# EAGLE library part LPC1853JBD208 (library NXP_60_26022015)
32-bit ARM Cortex-M3 MCU; up to 1 MB flash and 136 kB SRAM; Ethernet, two High-speed USB, LCD, EMC The LPC185x/3x/2x/1x are ARM Cortex-M3 based microcontrollers for embedded applications. The ARM Cortex-M3 is a next generation core that offers system enhancements such as low power consumption, enhanced debug features, and a high level of support block integration. The LPC185x/3x/2x/1x operate at CPU frequencies of up to 180 MHz. The ARM Cortex-M3 CPU incorporates a 3-stage pipeline and uses a Harvard architecture with separate local instruction and data buses as well as a third bus for peripherals. The ARM Cortex-M3 CPU also includes an internal prefetch unit that supports speculative branching. The LPC185x/3x/2x/1x include up to 1 MB of flash and 136 kB of on-chip SRAM, 16 kB of EEPROM memory, a quad SPI Flash Interface (SPIFI), a State Configurable Timer (SCT) subsystem, two High-speed USB controllers, Ethernet, LCD, an external memory controller, and multiple digital and analog peripherals. AAL Eindhoven MK
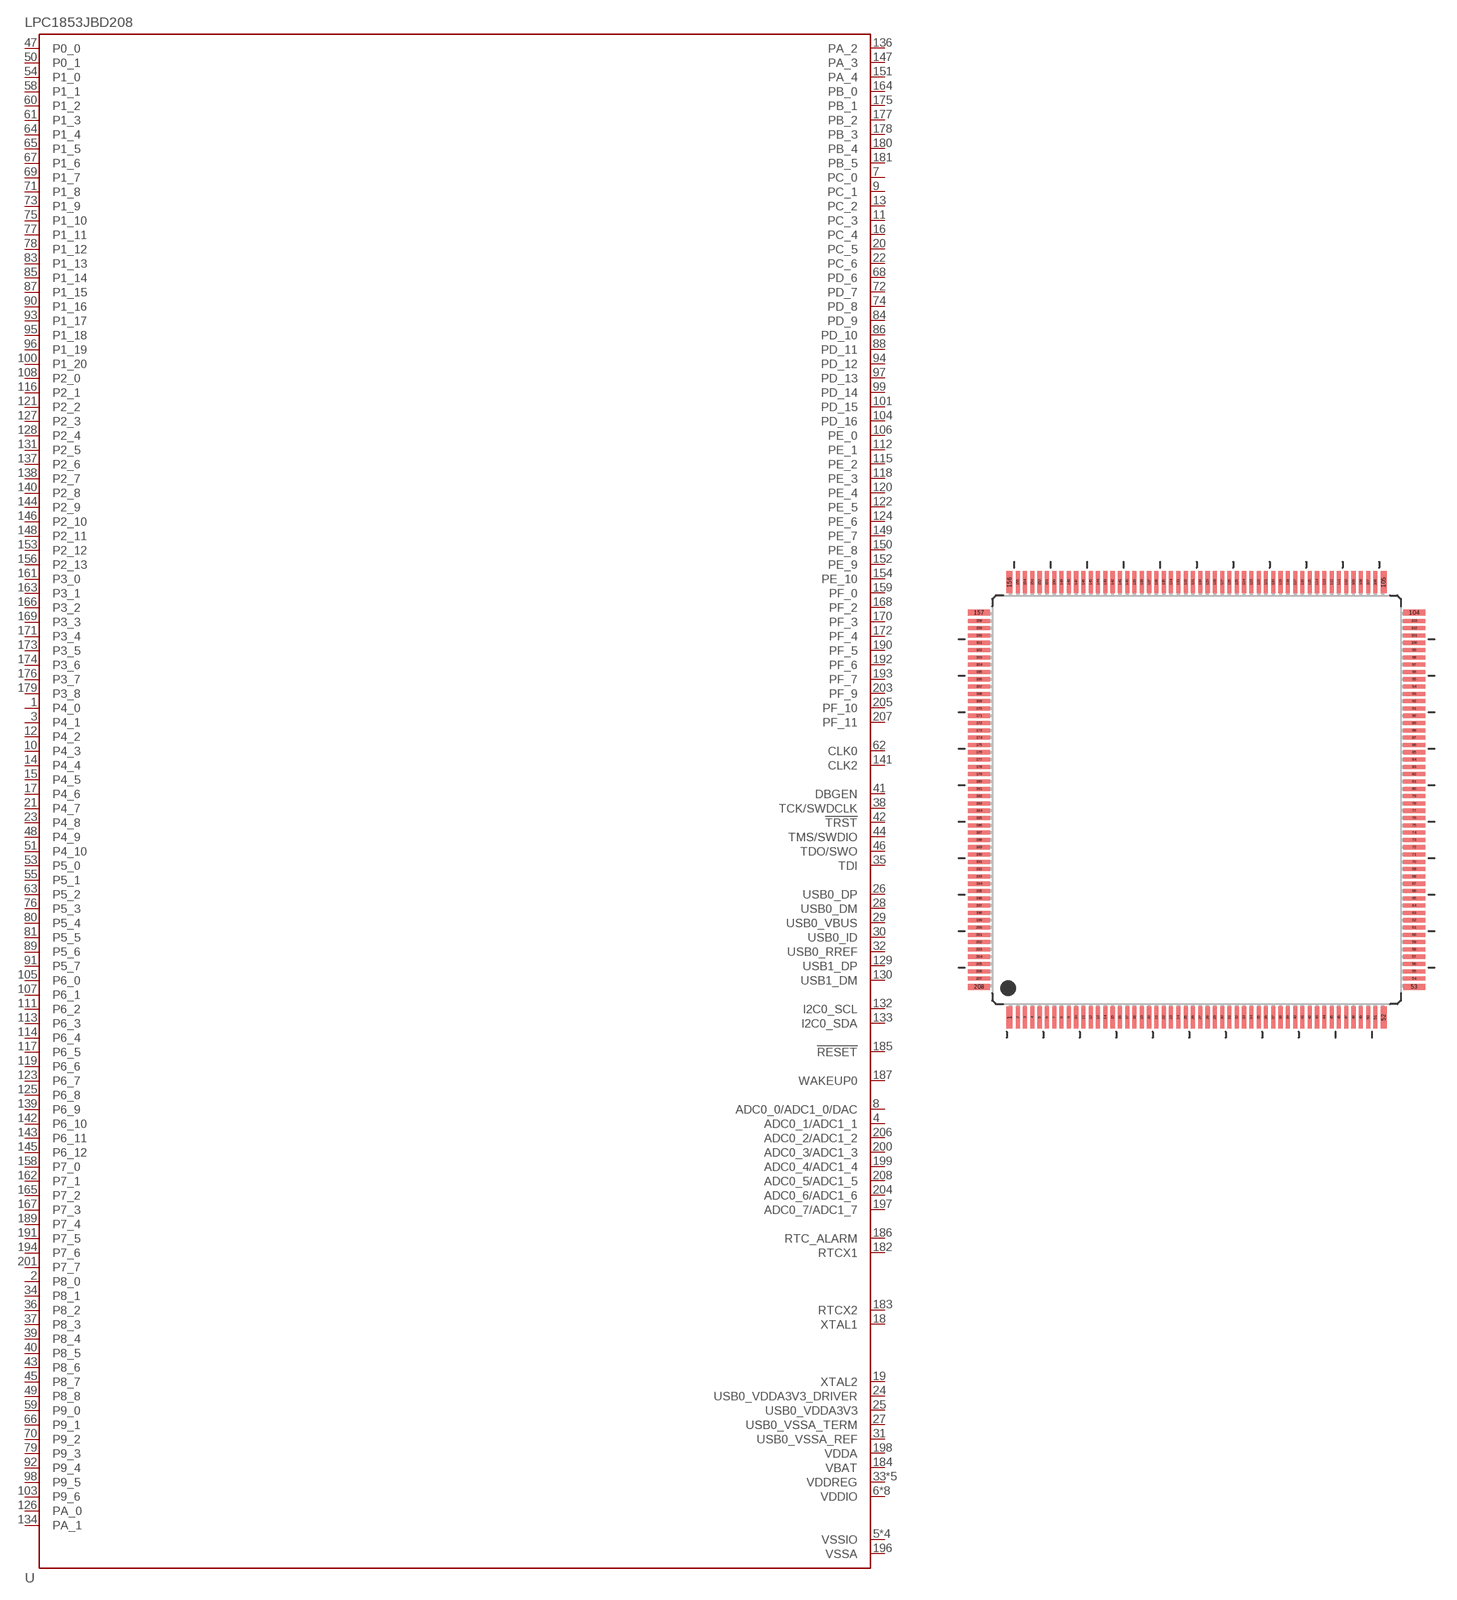
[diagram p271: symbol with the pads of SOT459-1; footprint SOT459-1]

Designator prefix U

## LPC1853JBD208 (ADC: 8; ETHERNET: yes; FLASH: 512kB; GPIO: 142; LCD: no; PWM: yes; QEI: yes; SRAM: 136kB; TEMPERATURE_RANGE: -40 °C to +105 °C; USB0: Host/OTG; USB1: Host/ULPI)  [SOT459-1]
1  P4_0
2  P8_0
3  P4_1
4  ADC0_1/ADC1_1
5  VSSIO
6  VDDIO
7  PC_0
8  ADC0_0/ADC1_0/DAC
9  PC_1
10  P4_3
11  PC_3
12  P4_2
13  PC_2
14  P4_4
15  P4_5
16  PC_4
17  P4_6
18  XTAL1
19  XTAL2
20  PC_5
21  P4_7
22  PC_6
23  P4_8
24  USB0_VDDA3V3_DRIVER
25  USB0_VDDA3V3
26  USB0_DP
27  USB0_VSSA_TERM
28  USB0_DM
29  USB0_VBUS
30  USB0_ID
31  USB0_VSSA_REF
32  USB0_RREF
33  VDDREG
34  P8_1
35  TDI
36  P8_2
37  P8_3
38  TCK/SWDCLK
39  P8_4
40  P8_5
41  DBGEN
42  !TRST
43  P8_6
44  TMS/SWDIO
45  P8_7
46  TDO/SWO
47  P0_0
48  P4_9
49  P8_8
50  P0_1
51  P4_10
52  VDDIO
53  P5_0
54  P1_0
55  P5_1
56  VSSIO
57  VDDIO
58  P1_1
59  P9_0
60  P1_2
61  P1_3
62  CLK0
63  P5_2
64  P1_4
65  P1_5
66  P9_1
67  P1_6
68  PD_6
69  P1_7
70  P9_2
71  P1_8
72  PD_7
73  P1_9
74  PD_8
75  P1_10
76  P5_3
77  P1_11
78  P1_12
79  P9_3
80  P5_4
81  P5_5
82  VDDREG
83  P1_13
84  PD_9
85  P1_14
86  PD_10
87  P1_15
88  PD_11
89  P5_6
90  P1_16
91  P5_7
92  P9_4
93  P1_17
94  PD_12
95  P1_18
96  P1_19
97  PD_13
98  P9_5
99  PD_14
100  P1_20
101  PD_15
102  VDDIO
103  P9_6
104  PD_16
105  P6_0
106  PE_0
107  P6_1
108  P2_0
109  VSSIO
110  VDDIO
111  P6_2
112  PE_1
113  P6_3
114  P6_4
115  PE_2
116  P2_1
117  P6_5
118  PE_3
119  P6_6
120  PE_4
121  P2_2
122  PE_5
123  P6_7
124  PE_6
125  P6_8
126  PA_0
127  P2_3
128  P2_4
129  USB1_DP
130  USB1_DM
131  P2_5
132  I2C0_SCL
133  I2C0_SDA
134  PA_1
135  VDDREG
136  PA_2
137  P2_6
138  P2_7
139  P6_9
140  P2_8
141  CLK2
142  P6_10
143  P6_11
144  P2_9
145  P6_12
146  P2_10
147  PA_3
148  P2_11
149  PE_7
150  PE_8
151  PA_4
152  PE_9
153  P2_12
154  PE_10
155  VDDIO
156  P2_13
157  VSSIO
158  P7_0
159  PF_0
160  VDDIO
161  P3_0
162  P7_1
163  P3_1
164  PB_0
165  P7_2
166  P3_2
167  P7_3
168  PF_2
169  P3_3
170  PF_3
171  P3_4
172  PF_4
173  P3_5
174  P3_6
175  PB_1
176  P3_7
177  PB_2
178  PB_3
179  P3_8
180  PB_4
181  PB_5
182  RTCX1
183  RTCX2
184  VBAT
185  !RESET
186  RTC_ALARM
187  WAKEUP0
188  VDDREG
189  P7_4
190  PF_5
191  P7_5
192  PF_6
193  PF_7
194  P7_6
195  VDDREG
196  VSSA
197  ADC0_7/ADC1_7
198  VDDA
199  ADC0_4/ADC1_4
200  ADC0_3/ADC1_3
201  P7_7
202  VDDIO
203  PF_9
204  ADC0_6/ADC1_6
205  PF_10
206  ADC0_2/ADC1_2
207  PF_11
208  ADC0_5/ADC1_5

## Footprint SOT459-1 (pad centres in mm)
SOT459-1 LQFP208; plastic low profile quad flat package; 208 leads; body 28 x 28 x 1.4 mm JEDEC: MS-026 IEC: 136E30 JEITA: --
smd 0.4 x 1.5: 1 -12.81,-14.9; 52 12.81,-14.9; 105 12.81,14.9; 156 -12.81,14.9
smd 0.28 x 1.5: 2 -12.25,-14.9; 3 -11.75,-14.9; 4 -11.25,-14.9; 5 -10.75,-14.9; 6 -10.25,-14.9; 7 -9.75,-14.9; 8 -9.25,-14.9; 9 -8.75,-14.9; 10 -8.25,-14.9; 11 -7.75,-14.9; 12 -7.25,-14.9; 13 -6.75,-14.9; 14 -6.25,-14.9; 15 -5.75,-14.9; 16 -5.25,-14.9; 17 -4.75,-14.9; 18 -4.25,-14.9; 19 -3.75,-14.9; 20 -3.25,-14.9; 21 -2.75,-14.9; 22 -2.25,-14.9; 23 -1.75,-14.9; 24 -1.25,-14.9; 25 -0.75,-14.9; 26 -0.25,-14.9; 27 0.25,-14.9; 28 0.75,-14.9; 29 1.25,-14.9; 30 1.75,-14.9; 31 2.25,-14.9; 32 2.75,-14.9; 33 3.25,-14.9; 34 3.75,-14.9; 35 4.25,-14.9; 36 4.75,-14.9; 37 5.25,-14.9; 38 5.75,-14.9; 39 6.25,-14.9; 40 6.75,-14.9; 41 7.25,-14.9; 42 7.75,-14.9; 43 8.25,-14.9; 44 8.75,-14.9; 45 9.25,-14.9; 46 9.75,-14.9; 47 10.25,-14.9; 48 10.75,-14.9; 49 11.25,-14.9; 50 11.75,-14.9; 51 12.25,-14.9; 106 12.25,14.9; 107 11.75,14.9; 108 11.25,14.9; 109 10.75,14.9; 110 10.25,14.9; 111 9.75,14.9; 112 9.25,14.9; 113 8.75,14.9; 114 8.25,14.9; 115 7.75,14.9; 116 7.25,14.9; 117 6.75,14.9; 118 6.25,14.9; 119 5.75,14.9; 120 5.25,14.9; 121 4.75,14.9; 122 4.25,14.9; 123 3.75,14.9; 124 3.25,14.9; 125 2.75,14.9; 126 2.25,14.9; 127 1.75,14.9; 128 1.25,14.9; 129 0.75,14.9; 130 0.25,14.9; 131 -0.25,14.9; 132 -0.75,14.9; 133 -1.25,14.9; 134 -1.75,14.9; 135 -2.25,14.9; 136 -2.75,14.9; 137 -3.25,14.9; 138 -3.75,14.9; 139 -4.25,14.9; 140 -4.75,14.9; 141 -5.25,14.9; 142 -5.75,14.9; 143 -6.25,14.9; 144 -6.75,14.9; 145 -7.25,14.9; 146 -7.75,14.9; 147 -8.25,14.9; 148 -8.75,14.9; 149 -9.25,14.9; 150 -9.75,14.9; 151 -10.25,14.9; 152 -10.75,14.9; 153 -11.25,14.9; 154 -11.75,14.9; 155 -12.25,14.9
smd 1.5 x 0.4: 53 14.9,-12.81; 104 14.9,12.81; 157 -14.9,12.81; 208 -14.9,-12.81
smd 1.5 x 0.28: 54 14.9,-12.25; 55 14.9,-11.75; 56 14.9,-11.25; 57 14.9,-10.75; 58 14.9,-10.25; 59 14.9,-9.75; 60 14.9,-9.25; 61 14.9,-8.75; 62 14.9,-8.25; 63 14.9,-7.75; 64 14.9,-7.25; 65 14.9,-6.75; 66 14.9,-6.25; 67 14.9,-5.75; 68 14.9,-5.25; 69 14.9,-4.75; 70 14.9,-4.25; 71 14.9,-3.75; 72 14.9,-3.25; 73 14.9,-2.75; 74 14.9,-2.25; 75 14.9,-1.75; 76 14.9,-1.25; 77 14.9,-0.75; 78 14.9,-0.25; 79 14.9,0.25; 80 14.9,0.75; 81 14.9,1.25; 82 14.9,1.75; 83 14.9,2.25; 84 14.9,2.75; 85 14.9,3.25; 86 14.9,3.75; 87 14.9,4.25; 88 14.9,4.75; 89 14.9,5.25; 90 14.9,5.75; 91 14.9,6.25; 92 14.9,6.75; 93 14.9,7.25; 94 14.9,7.75; 95 14.9,8.25; 96 14.9,8.75; 97 14.9,9.25; 98 14.9,9.75; 99 14.9,10.25; 100 14.9,10.75; 101 14.9,11.25; 102 14.9,11.75; 103 14.9,12.25; 158 -14.9,12.25; 159 -14.9,11.75; 160 -14.9,11.25; 161 -14.9,10.75; 162 -14.9,10.25; 163 -14.9,9.75; 164 -14.9,9.25; 165 -14.9,8.75; 166 -14.9,8.25; 167 -14.9,7.75; 168 -14.9,7.25; 169 -14.9,6.75; 170 -14.9,6.25; 171 -14.9,5.75; 172 -14.9,5.25; 173 -14.9,4.75; 174 -14.9,4.25; 175 -14.9,3.75; 176 -14.9,3.25; 177 -14.9,2.75; 178 -14.9,2.25; 179 -14.9,1.75; 180 -14.9,1.25; 181 -14.9,0.75; 182 -14.9,0.25; 183 -14.9,-0.25; 184 -14.9,-0.75; 185 -14.9,-1.25; 186 -14.9,-1.75; 187 -14.9,-2.25; 188 -14.9,-2.75; 189 -14.9,-3.25; 190 -14.9,-3.75; 191 -14.9,-4.25; 192 -14.9,-4.75; 193 -14.9,-5.25; 194 -14.9,-5.75; 195 -14.9,-6.25; 196 -14.9,-6.75; 197 -14.9,-7.25; 198 -14.9,-7.75; 199 -14.9,-8.25; 200 -14.9,-8.75; 201 -14.9,-9.25; 202 -14.9,-9.75; 203 -14.9,-10.25; 204 -14.9,-10.75; 205 -14.9,-11.25; 206 -14.9,-11.75; 207 -14.9,-12.25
